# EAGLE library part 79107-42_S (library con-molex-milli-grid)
RECEPTACAL
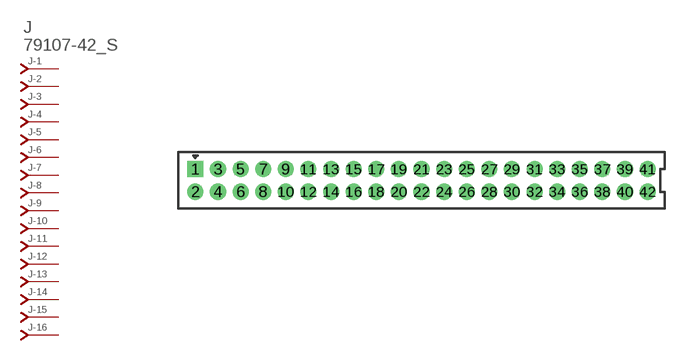
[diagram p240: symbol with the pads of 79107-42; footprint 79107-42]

Designator prefix J; gates -1=J-NV -2=J-N -3=J-N -4=J-N -5=J-N -6=J-N -7=J-N -8=J-N -9=J-N -10=J-N -11=J-N -12=J-N -13=J-N -14=J-N -15=J-N -16=J-N -17=J-N -18=J-N -19=J-N -20=J-N -21=J-N -22=J-N -23=J-N -24=J-N -25=J-N -26=J-N -27=J-N -28=J-N -29=J-N -30=J-N -31=J-N -32=J-N -33=J-N -34=J-N -35=J-N -36=J-N -37=J-N -38=J-N -39=J-N -40=J-N -41=J-N -42=J-N

## 79107-42_S  [79107-42]
1  -1:J  pas
2  -2:J  pas
3  -3:J  pas
4  -4:J  pas
5  -5:J  pas
6  -6:J  pas
7  -7:J  pas
8  -8:J  pas
9  -9:J  pas
10  -10:J  pas
11  -11:J  pas
12  -12:J  pas
13  -13:J  pas
14  -14:J  pas
15  -15:J  pas
16  -16:J  pas
17  -17:J  pas
18  -18:J  pas
19  -19:J  pas
20  -20:J  pas
21  -21:J  pas
22  -22:J  pas
23  -23:J  pas
24  -24:J  pas
25  -25:J  pas
26  -26:J  pas
27  -27:J  pas
28  -28:J  pas
29  -29:J  pas
30  -30:J  pas
31  -31:J  pas
32  -32:J  pas
33  -33:J  pas
34  -34:J  pas
35  -35:J  pas
36  -36:J  pas
37  -37:J  pas
38  -38:J  pas
39  -39:J  pas
40  -40:J  pas
41  -41:J  pas
42  -42:J  pas

## Footprint 79107-42 (pad centres in mm)
RECEPTACAL Dual Row, Vertical, Through-Hole
drill 0.914 square: 1 -20,1
drill 0.914: 2 -20,-1; 3 -18,1; 4 -18,-1; 5 -16,1; 6 -16,-1; 7 -14,1; 8 -14,-1; 9 -12,1; 10 -12,-1; 11 -10,1; 12 -10,-1; 13 -8,1; 14 -8,-1; 15 -6,1; 16 -6,-1; 17 -4,1; 18 -4,-1; 19 -2,1; 20 -2,-1; 21 0,1; 22 0,-1; 23 2,1; 24 2,-1; 25 4,1; 26 4,-1; 27 6,1; 28 6,-1; 29 8,1; 30 8,-1; 31 10,1; 32 10,-1; 33 12,1; 34 12,-1; 35 14,1; 36 14,-1; 37 16,1; 38 16,-1; 39 18,1; 40 18,-1; 41 20,1; 42 20,-1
